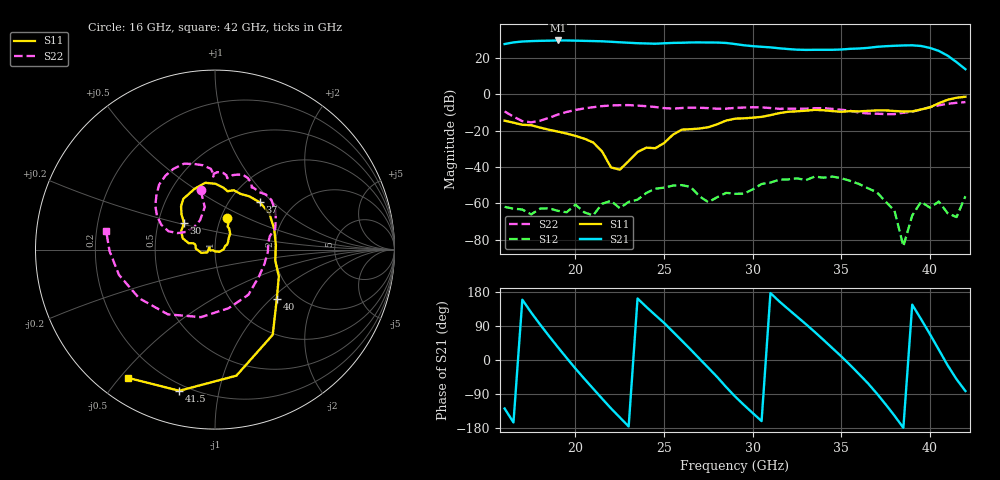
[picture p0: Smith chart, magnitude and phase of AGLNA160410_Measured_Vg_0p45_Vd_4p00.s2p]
! Filename4Jim: AG19_M062_CP1_C_1215_Vg_0p45_Vd_4p00_NF.s2p
! Calibration: TFN_AG02
! Notes: BK
! Row:12, Col:15
! Probes: GSG150
! Prober: TS150
! Date: 2024-01-23 11:25:53
! DC: Vg.V=0.452838, Vg.I=7.47036e-09, Vd.V=3.99986, Vd.I=0.0897444
! Keysight Technologies,N5245B,MY58421923,A.15.75.19
! AGMDC-PNAX50 Tue Jan 23 11:26:34 2024
# HZ S DB R 50
!freq (Hz)  S11DB  S11A  S21DB  S21A  S12DB  S12A  S22DB  S22A
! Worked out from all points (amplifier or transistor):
!   53 points, 16 GHz to 42 GHz, reference 50 ohm
!   highest |S21| = 29.7 dB at 19 GHz (marker M1)
!   |S21| within 3 dB of that: start of sweep to 29.86 GHz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
!   unconditionally stable (mu >= 1): start of sweep to end of sweep
!   at 20 GHz: K = 15.30, MAG = 30.3 dB, |S12| = -60.7 dB
!   at 29 GHz: K = 8.74, MAG = 28.8 dB, |S12| = -54.7 dB
!   at 42 GHz: K = 10.06, MAG = 22.0 dB, |S12| = -56.1 dB
!   lowest NFmin = 1.66 dB at 31.5 GHz
!   S11 on the Smith chart (normalised r, x): 16 GHz: 1.07, +0.39; 30 GHz: 0.68, +0.21; 37 GHz: 1.38, +0.83; 40 GHz: 1.59, -1.09; 41.5 GHz: 0.17, -0.77; 42 GHz: 0.09, -0.53
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1.6e10  -14.44 69.0  27.74 -128.0  -61.92 79.0  -9.39 103.6
1.7e10  -16.70 61.3  29.14 159.0  -63.38 77.5  -14.71 116.9
1.8e10  -18.25 46.1  29.52 93.8  -62.88 107.2  -14.48 148.5
1.9e10  -20.46 37.8  29.73 34.2  -64.11 115.5  -11.10 158.5
2.05e10  -24.36 19.9  29.50 -49.6  -64.97 103.8  -7.67 143.6
2.15e10  -31.39 -27.5  29.27 -101.9  -60.21 125.4  -6.43 130.8
2.25e10  -41.44 -121.4  28.73 -151.5  -62.66 105.7  -5.92 117.2
2.35e10  -31.74 -168.5  28.21 162.4  -57.97 134.8  -6.16 104.0
2.5e10  -26.76 -159.9  28.18 97.8  -51.32 105.0  -7.53 91.1
2.7e10  -18.77 165.0  28.65 3.2  -56.16 43.3  -7.34 84.0
2.9e10  -13.35 151.4  27.76 -96.1  -54.70 78.3  -7.41 76.7
3e10  -12.81 139.3  26.60 -140.0  -52.30 88.8  -7.03 69.8
3.15e10  -10.28 128.1  25.41 154.6  -46.92 50.4  -7.92 59.4
3.35e10  -8.49 98.3  24.58 74.0  -45.26 16.0  -7.58 47.2
3.55e10  -9.20 72.5  25.12 -13.5  -47.60 -41.2  -9.00 19.1
3.7e10  -8.80 46.4  26.22 -88.3  -53.86 -82.9  -10.61 -2.5
3.8e10  -9.13 19.4  26.79 -147.1  -64.08 -56.1  -10.82 -32.1
3.9e10  -9.35 -10.1  27.07 146.0  -66.66 5.2  -9.49 -76.8
4e10  -7.12 -38.6  25.63 68.2  -62.39 -19.2  -7.01 -126.1
4.05e10  -4.83 -55.9  23.98 27.1  -58.99 -47.2  -5.99 -147.3
4.15e10  -1.82 -104.2  17.79 -50.7  -67.55 101.9  -4.61 -179.2
4.2e10  -1.27 -124.2  13.91 -81.9  -56.06 44.5  -4.21 170.2
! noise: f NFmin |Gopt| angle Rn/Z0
1.6e+10  3.182  0.2371  -64.17  0.5202
1.85e+10  2.512  0.2009  -19.39  0.3818
2.15e+10  2.218  0  90  0.1666
2.45e+10  2.275  0.1313  67.44  0.4589
2.75e+10  2.38  0.05992  143.3  0.3905
3e+10  2.686  0.1172  35.71  1.204
3.3e+10  2.393  0  90  0.1838
3.6e+10  2.255  0  90  0.1702
3.9e+10  2.08  0  90  0.1535
4.2e+10  3.635  0  90  0.3274
